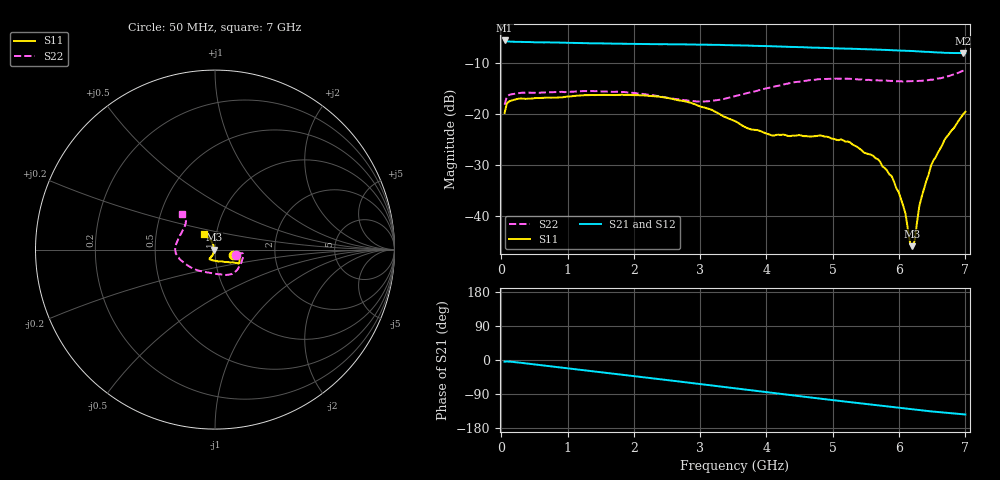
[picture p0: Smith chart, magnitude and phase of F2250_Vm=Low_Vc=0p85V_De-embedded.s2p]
! Integrated Device Technology
! Corporate Headquarters
! 6024 Silver Creek Valley Road
! San Jose, CA 95138  USA
! Phone:  1-408-284-8200
! Toll Free:  1-800-223-1366
! Webpage:  http://www.idt.com/
! Timing and RF Division
! 515 Groton Road, Suite 102
! Westford, MA 01886-6024
! Device:  F2250
! Description: Voltage Variable RF Attenuator
! Frequency:  50.0 -  6000.00 MHz
! Package:  3x3 mm Thin QFN Plastic Package: 16 pin
! Ports:  2 RF, 3 DC
!  Pin  1  = GND
!  Pin  2  = NC
!  Pin  3  = RF1  = Port 1
!  Pin  4  = NC
!  Pin  5  = GND
!  Pin  6  = GND
!  Pin  7  = GND
!  Pin  8  = GND
!  Pin  9  = NC
!  Pin 10  = RF2  = Port 2
!  Pin 11  = NC
!  Pin 12  = GND
!  Pin 13  = GND
!  Pin 14  = VCNTRL
!  Pin 15  = VDD
!  Pin 16  = VMODE
! Vcntrl:  0.850 Volts
! Vmode:  +0.000 Volts
! Vdd:  +3.30  Volts
! Current:  1.169 mA
! Data:  The device was measured on a the F2250 evaluation board which has
!  individual transmission lines to the RF pins.  Data was collected
!  using a calibrated network analyzer.  The evaluation board was
!  de-embedded using a TRL calibration technique.
!  The reference plane is the edge of the package pin.
! Misc:  SN 10
!  Action Tracker AT0258
! Date Measured:  2014-11-26
! Date:  2015-10-15  MJV
! Note:
!  Integrated Device Technology supplies this data as a sample of measured
!  data at the package pin for this product.  Your particular data for this
!  product may vary.
!  Data was taken at 25 degrees C.
!  Integrated Device Technology reserves the right to change this data at anytime.
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# GHz S dB R 50
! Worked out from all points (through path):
!   201 points, 50 MHz to 7 GHz, reference 50 ohm
!   highest |S21| = -5.58 dB at 50 MHz (marker M1); lowest = -8.1 dB at 6.965 GHz (marker M2)
!   group delay of S21, straight-line fit = 57.6 ps
!   lowest |S11| = -45.9 dB at 6.201 GHz (marker M3), VSWR 1.01, Z = 49.5 + j0.0484 ohm
!   |S11| at or under -10 dB: start of sweep to end of sweep
!   |S22| runs from -18.2 to -11.3 dB; largest |S21 - S12| = 0.0016
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0.05  -19.78 -16.2  -5.58 -4.4  -5.58 -4.4  -18.19 -13.4
0.08475  -17.91 -8.7  -5.74 -3.9  -5.75 -3.9  -16.55 -8.2
0.22375  -17.11 -7.5  -5.86 -6.0  -5.85 -5.9  -15.99 -10.1
1.2315  -16.34 -25.8  -6.09 -26.9  -6.09 -26.9  -15.51 -42.6
2.37825  -16.61 -31.1  -6.31 -50.3  -6.31 -50.3  -16.50 -70.0
3.0385  -18.67 -37.6  -6.41 -64.3  -6.41 -64.3  -17.57 -100.7
3.525  -21.39 -53.4  -6.54 -74.8  -6.53 -74.8  -16.50 -129.2
4.081  -24.21 -87.4  -6.73 -86.7  -6.71 -86.7  -14.73 -154.6
4.7065  -24.37 -117.2  -6.98 -99.8  -6.99 -99.8  -13.32 -172.7
5.2625  -25.58 -119.1  -7.20 -111.2  -7.19 -111.3  -13.09 174.7
5.6795  -28.89 -114.2  -7.35 -119.7  -7.37 -119.8  -13.41 164.3
5.85325  -31.87 -111.8  -7.47 -123.2  -7.47 -123.3  -13.51 159.7
6.06175  -38.01 -117.4  -7.57 -127.4  -7.58 -127.5  -13.64 153.3
6.0965  -39.56 -123.8  -7.59 -128.2  -7.60 -128.2  -13.60 152.3
6.166  -45.40 -142.0  -7.63 -129.5  -7.62 -129.6  -13.58 149.9
6.20075  -45.93 174.4  -7.65 -130.3  -7.65 -130.3  -13.55 148.7
6.2355  -44.82 136.7  -7.68 -130.9  -7.68 -130.9  -13.57 147.4
6.305  -38.05 119.6  -7.75 -132.2  -7.74 -132.3  -13.50 145.2
6.47875  -30.26 111.0  -7.85 -135.5  -7.85 -135.5  -13.26 140.1
6.68725  -25.02 113.0  -8.01 -138.9  -8.00 -138.9  -12.73 134.9
6.96525  -20.09 123.6  -8.08 -143.3  -8.07 -143.4  -11.53 133.6
7  -19.56 124.2  -8.08 -143.8  -8.07 -143.9  -11.34 133.1
